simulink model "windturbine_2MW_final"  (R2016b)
settings: Solver=VariableStepAuto  StartTime=0  StopTime=3600  RelTol=1e-3
undefined symbols (not defined in the file or in its folder): c1, c2, c3, c4, c5, c6, cp_nom, Generation, lambda_nom, P_wind_base, Pelec_base, Pnom, re_lib, speed_nom, Turbine, Wind, wind_base
libraries: simulink x1

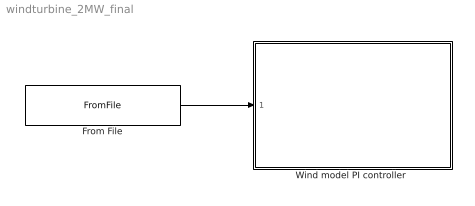
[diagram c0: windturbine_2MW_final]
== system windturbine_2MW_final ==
  From File : FromFile  FileName=windserie_test.mat  SampleTime=0
  "Wind model PI controller " : Subsystem
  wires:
  From File/1 -> "Wind model PI controller "/1("windspeed ")

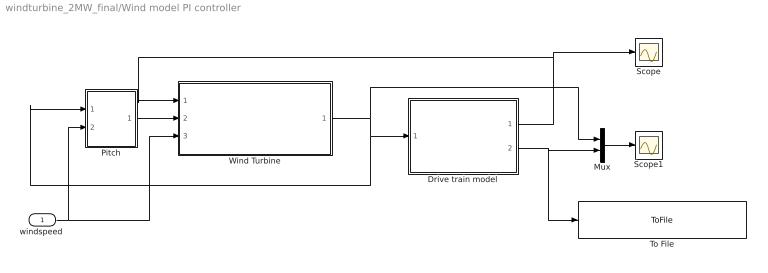
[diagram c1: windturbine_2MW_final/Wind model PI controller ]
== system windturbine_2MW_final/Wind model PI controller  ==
  "windspeed " : Inport
  Drive train model : Subsystem
  Mux : Mux  Inputs=2
  Pitch : Subsystem
  Scope : Scope
  Scope1 : Scope
  To File : ToFile  Commented=on  Filename=Pwt_moderate_windtest_2MW.mat  MatrixName=Pwt_moderate_windtest_6MW  SaveFormat=Timeseries
  Wind Turbine : Subsystem  AncestorBlock=re_lib/Wind Generation/Wind Turbine  DialogController=POWERSYS.PowerSysDialog
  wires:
  Drive train model/1(w) -> Scope/1, Wind Turbine/1(Generator speed (pu))
  Wind Turbine/1(Tm (pu)) -> Pitch/1(Tm), Drive train model/1(Tm), Mux/1
  "windspeed "/1 -> Wind Turbine/3(Wind speed (m/s)), Pitch/2(windspeed)
  Pitch/1(ß) -> Wind Turbine/2(Pitch angle (deg))
  Mux/1 -> Scope1/1
  Drive train model/2(Pe_ref) -> To File/1, Mux/2

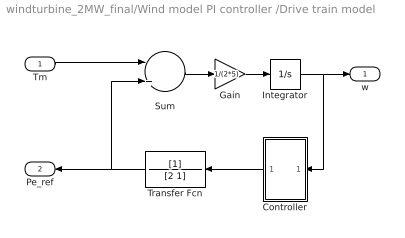
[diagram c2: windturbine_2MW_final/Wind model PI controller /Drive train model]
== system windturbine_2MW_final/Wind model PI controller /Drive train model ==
  Tm : Inport
  Controller : Subsystem
  Gain : Gain  Gain=1/(2*5)
  Integrator : Integrator  InitialCondition=1  LimitOutput=on  UpperSaturationLimit=2  LowerSaturationLimit=0
  Sum : Sum  Inputs=|+|-
  Transfer Fcn : TransferFcn  Denominator=[2 1]
  w : Outport
  Pe_ref : Outport  Port=2
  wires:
  Tm/1 -> Sum/1
  Sum/1 -> Gain/1
  Gain/1 -> Integrator/1
  Integrator/1 -> Controller/1(In1), w/1
  Transfer Fcn/1 -> Pe_ref/1, Sum/2
  Controller/1(Out1) -> Transfer Fcn/1

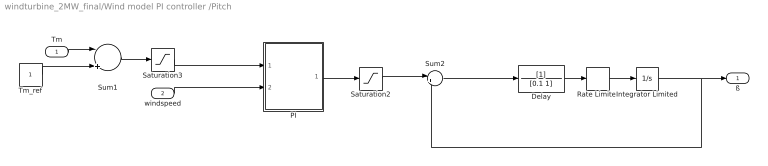
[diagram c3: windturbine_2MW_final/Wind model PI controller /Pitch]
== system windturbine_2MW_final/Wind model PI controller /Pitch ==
  Tm : Inport
  windspeed : Inport  Port=2
  Delay : TransferFcn  Denominator=[0.1 1]
  Integrator Limited : Integrator  LimitOutput=on  UpperSaturationLimit=90  LowerSaturationLimit=0
  PI : Subsystem
  Rate Limiter : RateLimiter  RisingSlewLimit=5  FallingSlewLimit=-5
  Saturation2 : Saturate  UpperLimit=90  LowerLimit=0  ZeroCross=off
  Saturation3 : Saturate  UpperLimit=1  LowerLimit=-1  ZeroCross=off
  Sum1 : Sum  Inputs=|+|-
  Sum2 : Sum  Inputs=|+-
  Tm_ref : Constant
  ß : Outport
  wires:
  Tm_ref/1 -> Sum1/2
  Delay/1 -> Rate Limiter/1
  Rate Limiter/1 -> Integrator Limited/1
  windspeed/1 -> PI/2(Wind speed)
  Saturation3/1 -> PI/1(∆Tm)
  PI/1(Out1) -> Saturation2/1
  Sum2/1 -> Delay/1
  Saturation2/1 -> Sum2/1
  Sum1/1 -> Saturation3/1
  Tm/1 -> Sum1/1
  Integrator Limited/1 -> Sum2/2, ß/1

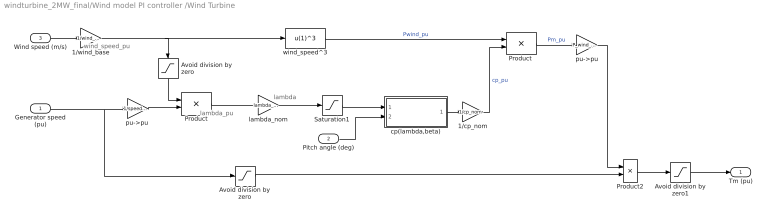
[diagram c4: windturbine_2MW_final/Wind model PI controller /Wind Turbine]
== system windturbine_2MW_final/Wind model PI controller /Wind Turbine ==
  note: wind_speed_pu
  note: lambda_pu
  note: lambda
  Generator speed (pu) : Inport
  Pitch angle (deg) : Inport  Port=2
  Wind speed (m/s) : Inport  Port=3
  1/cp_nom : Gain  Gain=1/cp_nom
  1/wind_base : Gain  Gain=1/wind_base
  Avoid division by zero : Saturate  UpperLimit=1e6  LowerLimit=1e-6
  "Avoid division by zero " : Saturate  UpperLimit=1e6  LowerLimit=1e-6
  Avoid division by zero1 : Saturate  UpperLimit=3  LowerLimit=0
  Product : Product  Inputs=/*
  "Product " : Product
  Product2 : Product  Inputs=*/
  Saturation1 : Saturate  UpperLimit=inf  LowerLimit=1e-6
  cp(lambda,beta) : Subsystem
  lambda_nom : Gain  Gain=lambda_nom
  pu->pu : Gain  Gain=P_wind_base*Pnom/Pelec_base
  "pu->pu " : Gain  Gain=1/speed_nom
  wind_speed^3 : Fcn  Expr=u(1)^3
  Tm (pu) : Outport
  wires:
  Pitch angle (deg)/1 -> cp(lambda,beta)/2(beta)
  pu->pu/1 -> Product2/1
  cp(lambda,beta)/1(cp) -> 1/cp_nom/1
  wind_speed^3/1 -> "Product "/1  "Pwind_pu"
  Avoid division by zero/1 -> Product2/2
  Wind speed (m/s)/1 -> 1/wind_base/1
  Generator speed (pu)/1 -> Avoid division by zero/1, "pu->pu "/1
  "Product "/1 -> pu->pu/1  "Pm_pu"
  lambda_nom/1 -> Saturation1/1
  1/cp_nom/1 -> "Product "/2  "cp_pu"
  Saturation1/1 -> cp(lambda,beta)/1(lambda)
  Product/1 -> lambda_nom/1
  1/wind_base/1 -> wind_speed^3/1, "Avoid division by zero "/1
  "Avoid division by zero "/1 -> Product/1
  "pu->pu "/1 -> Product/2
  Product2/1 -> Avoid division by zero1/1
  Avoid division by zero1/1 -> Tm (pu)/1

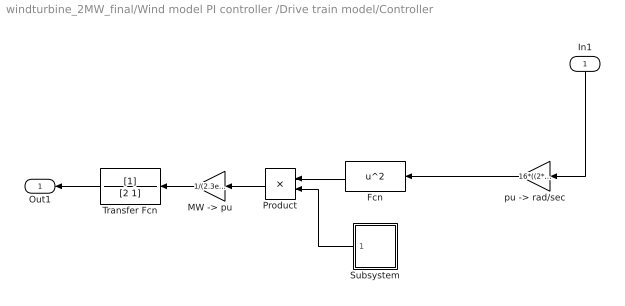
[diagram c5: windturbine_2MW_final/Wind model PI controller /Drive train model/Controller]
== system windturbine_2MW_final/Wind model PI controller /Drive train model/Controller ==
  In1 : Inport
  Fcn : Fcn  Expr=u^2
  "MW -> pu" : Gain  Gain=1/(2.3e6)
  Product : Product
  Subsystem : Subsystem
  Transfer Fcn : TransferFcn  Denominator=[2 1]
  "pu -> rad/sec" : Gain  Gain=16*((2*3.14)/60)
  Out1 : Outport
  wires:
  In1/1 -> "pu -> rad/sec"/1
  Fcn/1 -> Product/1
  Subsystem/1(K-opt) -> Product/2
  Product/1 -> "MW -> pu"/1
  "pu -> rad/sec"/1 -> Fcn/1
  Transfer Fcn/1 -> Out1/1
  "MW -> pu"/1 -> Transfer Fcn/1

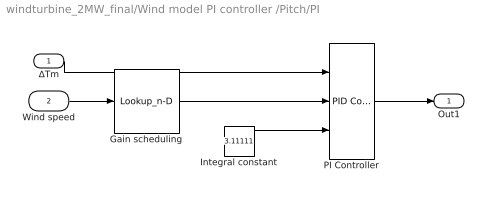
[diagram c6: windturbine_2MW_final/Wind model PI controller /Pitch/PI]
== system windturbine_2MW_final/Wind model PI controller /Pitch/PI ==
  ∆Tm : Inport
  Wind speed : Inport  Port=2
  Gain scheduling : Lookup_n-D  NumberOfTableDimensions=1  BreakpointsForDimension1=[10,12,14,15,16,17,18,19,20,21,22,23,24,25]  Table=[20,20,20,20,20,20,20,20,15,15,15,15,15,15]  InternalRulePriority=Speed  RndMeth=Simplest
  Integral constant : Constant  Value=3.11111
  PI Controller : simulink/Continuous/PID Controller  Controller=PI  TimeDomain=Continuous-time  SampleTime=-1  IntegratorMethod=Forward Euler  FilterMethod=Forward Euler  Form=Parallel  UseFilter=on  ControllerParametersSource=external  P=1  I=1  D=0  N=100  InitialConditionSource=internal  InitialConditionForIntegrator=0  InitialConditionForFilter=0  ExternalReset=none  LimitOutput=on  UpperSaturationLimit=90  LowerSaturationLimit=0  LinearizeAsGain=on  AntiWindupMode=clamping  Kb=1  TrackingMode=off  Kt=1  PParamMin=[]  PParamMax=[]  IParamMin=[]  IParamMax=[]  DParamMin=[]  DParamMax=[]  NParamMin=[]  NParamMax=[]  KbParamMin=[]  KbParamMax=[]  KtParamMin=[]  KtParamMax=[]  POutMin=[]  POutMax=[]  IOutMin=[0]  IOutMax=[]  DOutMin=[]  DOutMax=[]  NOutMin=[]  NOutMax=[]  KbOutMin=[]  KbOutMax=[]  KtOutMin=[]  KtOutMax=[]  IntegratorOutMin=[]  IntegratorOutMax=[]  FilterOutMin=[]  FilterOutMax=[]  SumOutMin=[]  SumOutMax=[]  SumI1OutMin=[]  SumI1OutMax=[]  SumI2OutMin=[]  SumI2OutMax=[]  SumI3OutMin=[]  SumI3OutMax=[]  SumDOutMin=[]  SumDOutMax=[]  SaturationOutMin=[]  SaturationOutMax=[]  IntegratorContinuousStateAttributes=''  IntegratorStateMustResolveToSignalObject=off  IntegratorRTWStateStorageClass=Auto  FilterContinuousStateAttributes=''  FilterStateMustResolveToSignalObject=off  FilterRTWStateStorageClass=Auto  DifferentiatorICPrevScaledInput=0  DifferentiatorOutMin=[]  DifferentiatorOutMax=[]
  Out1 : Outport
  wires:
  Gain scheduling/1 -> PI Controller/2
  Wind speed/1 -> Gain scheduling/1
  ∆Tm/1 -> PI Controller/1
  PI Controller/1 -> Out1/1
  Integral constant/1 -> PI Controller/3

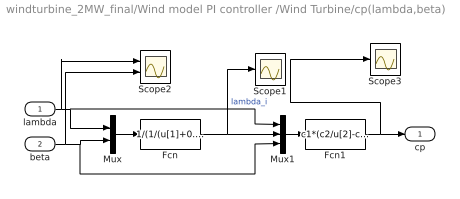
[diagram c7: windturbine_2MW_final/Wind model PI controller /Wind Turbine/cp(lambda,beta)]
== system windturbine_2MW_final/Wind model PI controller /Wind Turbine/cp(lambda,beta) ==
  lambda : Inport
  beta : Inport  Port=2
  Fcn : Fcn  Expr=1/(1/(u[1]+0.08*u[2])-0.035/(u[2]^3+1))
  Fcn1 : Fcn  Expr=c1*(c2/u[2]-c3*u[3]-c4)*exp(-c5/u[2])+c6*u[1]
  Mux : Mux  Inputs=2
  Mux1 : Mux  Inputs=3
  Scope1 : Scope
  Scope2 : Scope  NumInputPorts=2
  Scope3 : Scope
  cp : Outport
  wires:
  Fcn/1 -> Scope1/1, Mux1/2  "lambda_i"
  Fcn1/1 -> Scope3/1, cp/1
  lambda/1 -> Scope2/1, Mux1/1, Mux/1
  Mux1/1 -> Fcn1/1
  beta/1 -> Scope2/2, Mux1/3, Mux/2
  Mux/1 -> Fcn/1

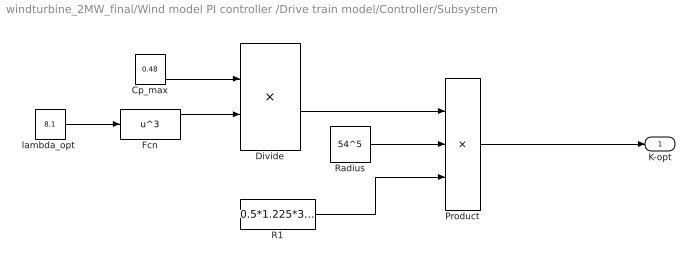
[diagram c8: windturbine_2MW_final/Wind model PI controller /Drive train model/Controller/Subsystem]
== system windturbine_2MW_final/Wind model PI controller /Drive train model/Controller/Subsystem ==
  Cp_max : Constant  Value=0.48
  Divide : Product  Inputs=*/
  Fcn : Fcn  Expr=u^3
  Product : Product  Inputs=3
  R1 : Constant  Value=0.5*1.225*3.14
  Radius : Constant  Value=54^5
  "lambda_opt " : Constant  Value=8.1
  K-opt : Outport
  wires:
  Divide/1 -> Product/1
  Radius/1 -> Product/2
  R1/1 -> Product/3
  Fcn/1 -> Divide/2
  "lambda_opt "/1 -> Fcn/1
  Cp_max/1 -> Divide/1
  Product/1 -> K-opt/1
